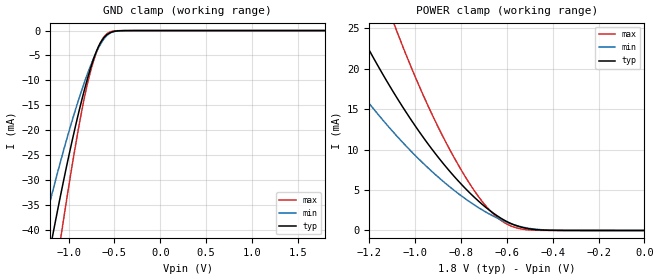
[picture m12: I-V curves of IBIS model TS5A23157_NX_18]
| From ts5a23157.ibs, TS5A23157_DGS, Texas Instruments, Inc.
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[Model]   TS5A23157_NX_18
Model_type  Terminator
| variable   typ   min   max
C_comp   6.17pF   5.48pF   6.61pF
| C_tri-state   6.17pF   5.48pF   6.61pF
[Temperature Range]   40   100   -40
| Ambient temperature   25   85   -40
[Voltage range]   1.8   1.65   1.95
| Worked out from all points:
|   GND clamp passes 1 mA (typ) near -0.59 V on its own axis
|   POWER clamp passes 1 mA (typ) near -0.59 V on its own axis
[GND Clamp]
| TS5A23157_NX_18
|   Voltage   I(typ)   I(min)   I(max)
-1.8V     -109mA     -83.84mA   -139.9mA
-1.28V    -51.6mA    -40.1mA    -66.49mA
-1.175V   -41.24mA   -32.35mA   -52.79mA
-1.155V   -39.33mA   -30.93mA   -50.24mA
-1.075V   -31.92mA   -25.4mA    -40.32mA
-905mV    -17.6mA    -14.69mA   -20.97mA
-790mV    -9.373mA   -8.461mA   -10.3mA
-735mV    -6.082mA   -5.888mA   -6.523mA
-670mV    -3.057mA   -3.322mA   -3.136mA
-565mV    -608.6uA   -733.8uA   -429.9uA
-390mV    -8.913uA   -13.04uA   -1.564uA
1.8V      85.24pA    48.31nA    15.28pA
[POWER Clamp]
| TS5A23157_NX_18
|   Voltage   I(typ)   I(min)   I(max)
-1.8V     61.46mA    42.96mA    95.88mA
-1.435V   35.72mA    24.96mA    55.6mA
-1.255V   25.16mA    17.68mA    38.73mA
-1.24V    24.36mA    17.12mA    37.43mA
-1.08V    16.41mA    11.67mA    24.62mA
-960mV    11.32mA    8.167mA    16.41mA
-835mV    6.847mA    5.071mA    9.259mA
-725mV    3.663mA    2.844mA    4.235mA
-635mV    1.677mA    1.439mA    1.451mA
-560mV    609.4uA    628.1uA    333.6uA
-475mV    111.3uA    156.6uA    29.51uA
-16.28fV  85.24pA    696.8pA    18.25pA
